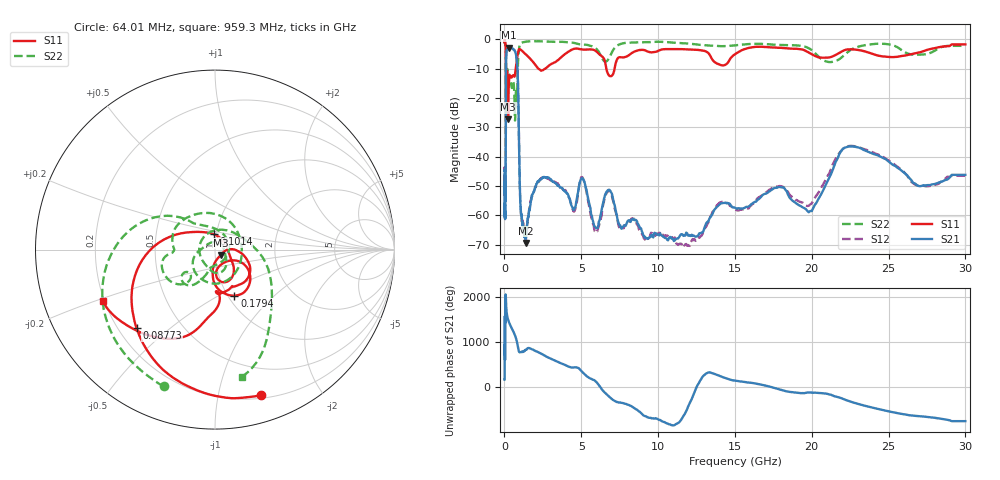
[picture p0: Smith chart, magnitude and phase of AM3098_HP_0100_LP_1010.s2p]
! Date/Time: Thu, Feb 28, 2019 8:35 AM
! Network Analyzer: Agilent Technologies E8364B Rev: A.07.50.67
! Sweep from 0.010 to 30.000 GHz, 1601 Points, Sweep Type: LOG
! Power Supply: 5.022 V, 0.002 A
# Hz S DB R 50
!freq MagS11 AngS11 MagS21 AngS21 MagS12 AngS12 MagS22 AngS22
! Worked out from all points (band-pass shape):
!   1601 points, 10 MHz to 30 GHz, reference 50 ohm
!   highest |S21| = -2.80 dB at 271.8 MHz (marker M1); lowest = -69.4 dB at 1.382 GHz (marker M2)
!   |S21| within 3 dB of the highest: 112 MHz to 772.4 MHz (660.4 MHz wide, 149 % of centre)
!   lowest |S11| = -27.3 dB at 236.3 MHz (marker M3), VSWR 1.09, Z = 53.2 - j3.11 ohm
!   |S11| at or under -10 dB: 95.95 MHz to 730.9 MHz (634.9 MHz wide, 154 % of centre); 2.224 GHz to 2.643 GHz (419.3 MHz wide, 17.2 % of centre); 6.633 GHz to 7.167 GHz (534.5 MHz wide, 7.75 % of centre)
!   |S22| runs from -27.6 to -0.6 dB; largest |S21 - S12| = 0.011
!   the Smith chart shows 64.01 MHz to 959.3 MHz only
!   S11 on the Smith chart (normalised r, x): 64.01 MHz: 0.23, -1.34; 87.73 MHz: 0.27, -0.39; 101.4 MHz: 0.97, +0.17; 179.4 MHz: 1.07, -0.60; 959.3 MHz: 0.19, -0.21
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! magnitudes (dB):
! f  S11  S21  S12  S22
! 10 MHz  -0.3  -44.8  -45.6  -0.6
! 38.04 MHz  -0.5  -59.0  -60.1  -0.9
! 64.01 MHz  -1.4  -51.4  -53.2  -1.8
! 76.65 MHz  -2.1  -54.8  -53.0  -2.6
! 87.73 MHz  -4.2  -34.2  -34.0  -4.6
! 101.4 MHz  -21.3  -10.1  -10.1  -22.4
! 144.7 MHz  -16.9  -3.6  -3.6  -13.6
! 179.4 MHz  -11.1  -3.3  -3.3  -10.0
! 236.3 MHz  -27.3  -2.9  -2.9  -12.5
! 271.8 MHz  -17.0  -2.8  -2.8  -12.8
! 550.5 MHz  -12.2  -3.3  -3.2  -14.6
! 825.6 MHz  -6.3  -8.5  -8.5  -17.9
! 959.3 MHz  -3.2  -38.8  -38.7  -2.8
! 1.082 GHz  -3.6  -59.5  -60.3  -1.2
! 1.382 GHz  -5.0  -69.4  -65.8  -0.7
! 2.084 GHz  -9.2  -49.4  -49.6  -0.6
! 5.077 GHz  -3.4  -47.4  -47.1  -1.7
! 7.926 GHz  -5.9  -63.1  -63.4  -1.1
! 12.07 GHz  -3.4  -67.0  -70.4  -1.4
! 19.8 GHz  -4.5  -59.0  -56.8  -3.0
! 22.67 GHz  -3.4  -36.5  -36.3  -3.2
! 30 GHz  -1.7  -46.2  -46.5  -2.2
